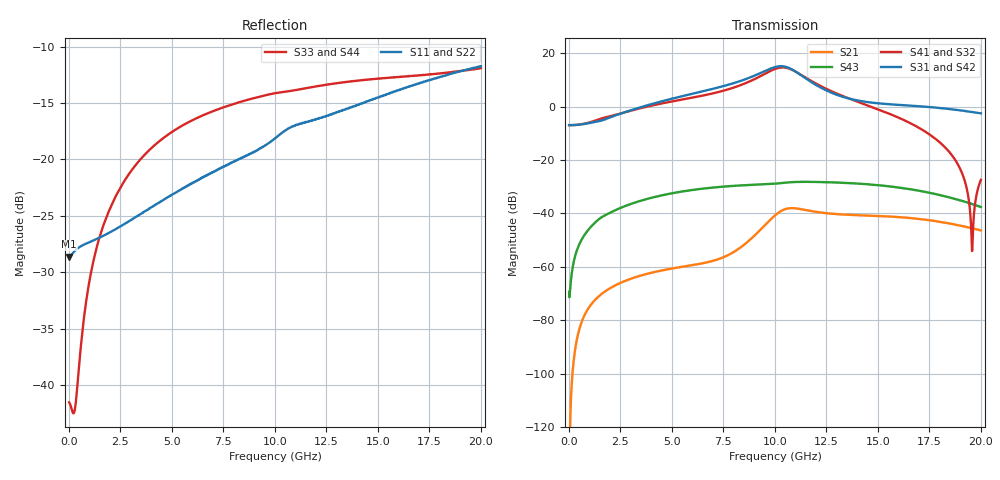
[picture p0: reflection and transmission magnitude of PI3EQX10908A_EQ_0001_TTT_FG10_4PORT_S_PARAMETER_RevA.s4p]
! NPort=4 DATA=2000 NOISE=0 GROUPDELAY=0 COMPLEX_DATAFORMAT=POLAR
! NumOfBlock=1 NumOfParam=0
! .MODEL Smodel S TSTONEFILE=PI3EQX10908A_EQ_0001_TTT_FG10_4PORT_S_PARAMETER_RevA.s4p TYPE=S
!  -- The above .MODEL line can be used for the S element in the netlist.
! The s parameter is extracted from the linear redriver, it is not bi-directional; only s(4,1)s(4,2) and s(3,1)s(3,2)
! should be the insertion loss
!Port definition:
!Port1 = input+
!Port2 = input-
!Port3 = output+
!Port4 = output-
# Hz S MA R  50
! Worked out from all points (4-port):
!   2000 points, 10 MHz to 20 GHz, reference 50 ohm
!   strongest paths, dB at 10 MHz, 5.01 GHz, 10.01 GHz, 15.01 GHz, 20 GHz:
!     S31: -6.9, 3.0, 14.8, 1.2, -2.5
!     S42: -6.9, 3.0, 14.8, 1.2, -2.5
!     S41: -6.9, 1.9, 14.1, -1.0, -27.4
!     S32: -6.9, 1.9, 14.1, -1.0, -27.5
!     S43: -69.4, -32.4, -28.9, -29.4, -37.6
!     S21: -127.3, -60.6, -40.7, -40.9, -46.4
!   lowest |S11| = -28.6 dB at 10 MHz (marker M1), VSWR 1.08, Z = 46.4 - j0.024 ohm
!   |S11| at or under -10 dB: start of sweep to end of sweep
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1e7  0.03701 -179.6  4.327e-07 13.5  0 0.0  0 0.0
     4.327e-07 13.5  0.03701 -179.6  0 0.0  0 0.0
     0.4502 -0.1  0.4502 179.9  0.008374 26.0  0.00034 -27.1
     0.4502 179.9  0.4502 -0.1  0.00034 -27.1  0.008374 26.0
7.94e9  0.09709 -117.3  0.001834 126.5  1.138e-06 51.5  4.259e-07 132.1
        0.001835 126.5  0.09713 -117.3  4.259e-07 132.1  1.138e-06 51.5
        2.706 -51.3  2.231 121.8  0.1756 2.2  0.03271 3.6
        2.231 121.8  2.706 -51.3  0.03271 3.6  0.1756 2.2
9.9e9  0.1221 -110.5  0.008446 120.3  5.15e-06 4.0  3.209e-06 123.5
       0.008445 120.3  0.1221 -110.5  3.208e-06 123.5  5.15e-06 4.0
       5.337 -108.3  4.875 66.3  0.1958 -12.1  0.03581 -15.1
       4.874 66.3  5.336 -108.3  0.03581 -15.1  0.1958 -12.1
1.067e10  0.1375 -111.0  0.01245 82.1  6.34e-06 -30.0  6.754e-06 85.1
          0.01245 82.1  0.1375 -111.0  6.753e-06 85.1  6.339e-06 -30.0
          5.326 -154.8  5.18 17.6  0.2009 -17.1  0.03816 -23.1
          5.18 17.6  5.326 -154.8  0.03816 -23.1  0.2009 -17.1
1.181e10  0.1485 -112.4  0.01099 42.6  5.928e-06 -37.0  9.975e-06 39.3
          0.011 42.6  0.1486 -112.4  9.973e-06 39.3  5.928e-06 -37.0
          2.811 162.5  2.959 -32.5  0.2094 -23.2  0.03896 -38.2
          2.959 -32.5  2.811 162.5  0.03896 -38.2  0.2094 -23.2
1.476e10  0.1852 -110.6  0.009042 2.8  2.289e-05 -54.6  2.472e-05 -26.0
          0.009048 2.7  0.1853 -110.6  2.472e-05 -26.0  2.29e-05 -54.6
          1.18 137.8  0.9653 -91.0  0.2271 -37.5  0.0345 -74.4
          0.9655 -91.0  1.18 137.8  0.0345 -74.4  0.2271 -37.5
2e10  0.2593 -113.8  0.004802 -51.3  9.234e-05 -148.0  7.206e-05 -136.6
      0.004808 -51.5  0.2594 -113.8  7.205e-05 -136.6  9.234e-05 -148.0
      0.7483 64.3  0.04241 -13.8  0.254 -52.2  0.01318 -136.9
      0.04252 -13.4  0.7479 64.3  0.01318 -136.9  0.254 -52.2
